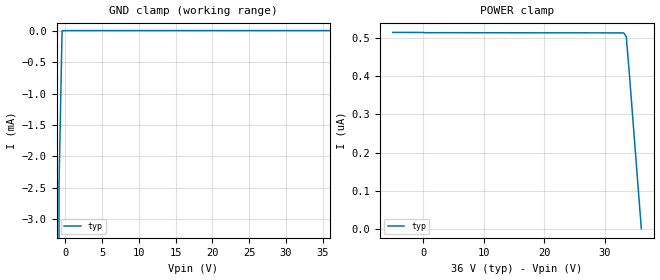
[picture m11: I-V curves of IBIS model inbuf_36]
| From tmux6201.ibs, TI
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| inbuf_36
[Model]   inbuf_36
Model_type   Input
Vinl = 0.8
Vinh = 1.3
|   typ   min   max
C_comp   4.014581e-13   NA   NA
[Voltage Range]   36   NA   NA
[Temperature Range]   27   NA   NA
[Power Clamp Reference]   36   NA   NA
[GND Clamp Reference]   0   NA   NA
[GND Clamp]
|   Voltage   I(typ)   I(min)   I(max)
-5V       -1.213A    NA         NA
-1.273V   -74.84mA   NA         NA
-858.6mV  -2.444mA   NA         NA
-444.4mV  -3.234uA   NA         NA
36V       515.5nA    NA         NA
[POWER Clamp]
|   Voltage   I(typ)   I(min)   I(max)
-5V       515.7nA    NA         NA
33.1V     514.2nA    NA         NA
33.52V    504.8nA    NA         NA
33.93V    426.7nA    NA         NA
36V       -195.4pA   NA         NA
